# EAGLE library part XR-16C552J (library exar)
DUAL UART with FIFO and parallel printer port
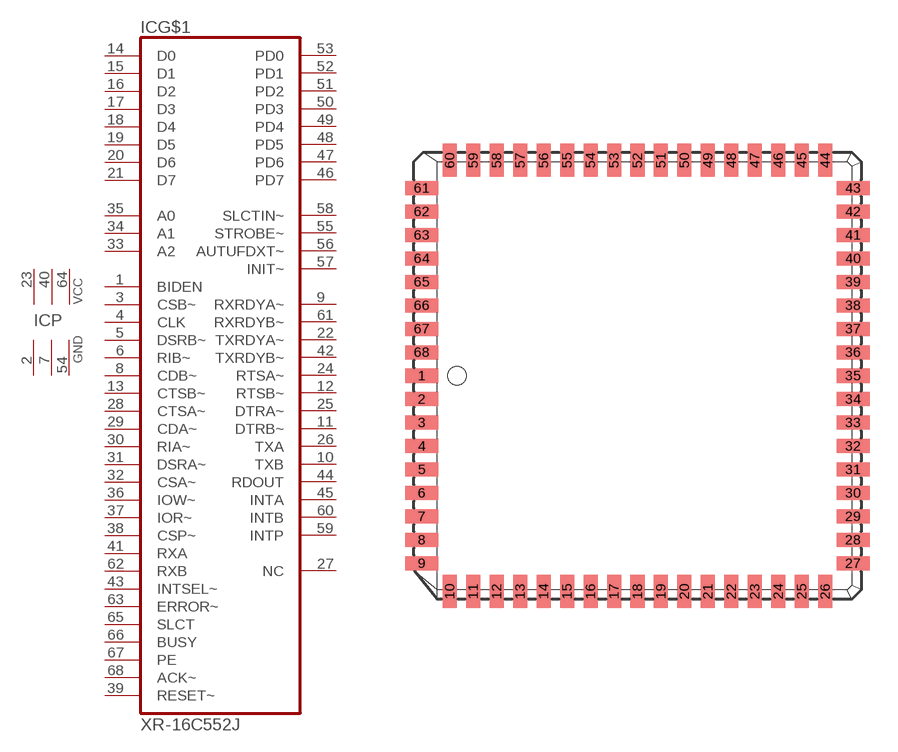
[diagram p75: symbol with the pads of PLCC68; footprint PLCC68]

Designator prefix IC; gates G$1=16C552J P=3VCC3GND

## XR-16C552J (MPN: TL16C552AFNRG4; OC_FARNELL: 1703245; OC_NEWARK: 99K4382)  [PLCC68]
1  G$1:BIDEN  in
2  P:GND  pwr
3  G$1:CSB~  in
4  G$1:CLK  in
5  G$1:DSRB~  in
6  G$1:RIB~  in
7  P:GND  pwr
8  G$1:CDB~  in
9  G$1:RXRDYA~  out
10  G$1:TXB  out
11  G$1:DTRB~  out
12  G$1:RTSB~  out
13  G$1:CTSB~  in
14  G$1:D0
15  G$1:D1
16  G$1:D2
17  G$1:D3
18  G$1:D4
19  G$1:D5
20  G$1:D6
21  G$1:D7
22  G$1:TXRDYA~  out
23  P:VCC  pwr
24  G$1:RTSA~  out
25  G$1:DTRA~  out
26  G$1:TXA  out
27  G$1:NC  nc
28  G$1:CTSA~  in
29  G$1:CDA~  in
30  G$1:RIA~  in
31  G$1:DSRA~  in
32  G$1:CSA~  in
33  G$1:A2  in
34  G$1:A1  in
35  G$1:A0  in
36  G$1:IOW~  in
37  G$1:IOR~  in
38  G$1:CSP~  in
39  G$1:RESET~  in
40  P:VCC  pwr
41  G$1:RXA  in
42  G$1:TXRDYB~  out
43  G$1:INTSEL~  in
44  G$1:RDOUT  out
45  G$1:INTA  out
46  G$1:PD7
47  G$1:PD6
48  G$1:PD5
49  G$1:PD4
50  G$1:PD3
51  G$1:PD2
52  G$1:PD1
53  G$1:PD0
54  P:GND  pwr
55  G$1:STROBE~
56  G$1:AUTUFDXT~
57  G$1:INIT~
58  G$1:SLCTIN~
59  G$1:INTP  out
60  G$1:INTB  out
61  G$1:RXRDYB~  out
62  G$1:RXB  in
63  G$1:ERROR~  in
64  P:VCC  pwr
65  G$1:SLCT  in
66  G$1:BUSY  in
67  G$1:PE  in
68  G$1:ACK~  in

## Footprint PLCC68 (pad centres in mm)
Plastic Leaded Chip Carrier
smd 1.8 x 0.76: 1 -11.67,0; 2 -11.67,-1.27; 3 -11.67,-2.54; 4 -11.67,-3.81; 5 -11.67,-5.08; 6 -11.67,-6.35; 7 -11.67,-7.62; 8 -11.67,-8.89; 9 -11.67,-10.16; 27 11.67,-10.16; 28 11.67,-8.89; 29 11.67,-7.62; 30 11.67,-6.35; 31 11.67,-5.08; 32 11.67,-3.81; 33 11.67,-2.54; 34 11.67,-1.27; 35 11.67,0; 36 11.67,1.27; 37 11.67,2.54; 38 11.67,3.81; 39 11.67,5.08; 40 11.67,6.35; 41 11.67,7.62; 42 11.67,8.89; 43 11.67,10.16; 61 -11.67,10.16; 62 -11.67,8.89; 63 -11.67,7.62; 64 -11.67,6.35; 65 -11.67,5.08; 66 -11.67,3.81; 67 -11.67,2.54; 68 -11.67,1.27
smd 0.76 x 1.8: 10 -10.16,-11.67; 11 -8.89,-11.67; 12 -7.62,-11.67; 13 -6.35,-11.67; 14 -5.08,-11.67; 15 -3.81,-11.67; 16 -2.54,-11.67; 17 -1.27,-11.67; 18 0,-11.67; 19 1.27,-11.67; 20 2.54,-11.67; 21 3.81,-11.67; 22 5.08,-11.67; 23 6.35,-11.67; 24 7.62,-11.67; 25 8.89,-11.67; 26 10.16,-11.67; 44 10.16,11.67; 45 8.89,11.67; 46 7.62,11.67; 47 6.35,11.67; 48 5.08,11.67; 49 3.81,11.67; 50 2.54,11.67; 51 1.27,11.67; 52 0,11.67; 53 -1.27,11.67; 54 -2.54,11.67; 55 -3.81,11.67; 56 -5.08,11.67; 57 -6.35,11.67; 58 -7.62,11.67; 59 -8.89,11.67; 60 -10.16,11.67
